(* Logix 5000 Rung export; software revision 16.05 *)

MODULES
   PBM : vendor None type None code None
   Local : vendor None type None code None
END_MODULES

TYPE ILX69PBM_STATUS_BACKPLANE :   // Backplane Block Status
STRUCT
   Input : ILX69PBM_STATUS_BACKPLANE_INPUT;
   Output : ILX69PBM_STATUS_BACKPLANE_OUTPUT;
END_STRUCT
END_TYPE

TYPE ILX69PBM_CONTROL_DPV1_WRITE_REQUEST :   // DPV1 Write Request
STRUCT
   Status : DINT;   // Status
   Command : DINT;   // Message Command. Set to 0x2212
   SlaveAddress : SINT;   // Slave Address
   SlotNumber : SINT;   // Slot Number
   Index : SINT;   // Index
   Length : SINT;   // Length
   Data : SINT[100];   // Write Data
END_STRUCT
END_TYPE

TYPE ILX69PBM_CONTROL_BACKPLANE :   // Backplane Block Control
STRUCT
   DisableAutoTransfer : BOOL;   // Disable Automatic Block Transfer
   Input : ILX69PBM_CONTROL_BACKPLANE_INPUT;
   Output : ILX69PBM_CONTROL_BACKPLANE_OUTPUT;
END_STRUCT
END_TYPE

TYPE ILX69PBM_UTIL_SLAVE_DIAG_COMMAND :   // Requested address for SlaveDiagnostic
STRUCT
   SlaveAddress : SINT;   // Slave Address
   DiagnosticMode : SINT;   // Diagnostic Mode
   Reserved1 : SINT;   // Reserved
   Reserved2 : SINT;   // Reserved
END_STRUCT
END_TYPE

TYPE ILX69PBM_CONTROL_BACKPLANE_OUTPUT :
STRUCT
   BlockID : SINT;   // Command Output Block Number. Use when DisableAutoTransfer is set.
   WriteBlock : BOOL;   // Send current commanded output block to module. Use when DisableAutoTransfer is set.
   CommitToProfibus : BOOL;   // Commit output block data to Profibus. Use when DisableAutoTransfer is set.
END_STRUCT
END_TYPE

TYPE ILX69PBM_UTIL_OUTPUT_ARRAY :
STRUCT
   DeviceCommandRegister : ILX69PBM_UTIL_DEV_COMMAND_REGISTER;   // Command Register
   DiagnosticSlaveAddress : ILX69PBM_UTIL_SLAVE_DIAG_COMMAND;   // Slave Address
   GlobalControlCommand : ILX69PBM_UTIL_GLOBAL_CONTROL_COMMAND;   // Global Control Command
   Reserved : SINT[4];   // Reserved
   OutputData : INT[240];   // PROFIBUS Output data.
END_STRUCT
END_TYPE

TYPE ILX69PBM_UTIL_GLOBAL_STATE_FIELD :   // PROFIBUS Master Global State Field
STRUCT
   ControlError : BOOL;   // Control error
   AutoClearError : BOOL;   // Auto clear error
   NonExchangeError : BOOL;   // Non exchange error
   FatalError : BOOL;   // Fatal error
   EventError : BOOL;   // Event error
   HostNotReady : BOOL;   // Host not ready notification
   Timeout : BOOL;   // Timeout
   Reserved1 : BOOL;   // Reserved
   MasterMainState : SINT;   // Master main state
   FaultySlaveAddress : SINT;   // Faulty remote address
   ErrorNumber : SINT;   // Error Number
   BusErrorCount : INT;   // Heavy bus error counter
   TimeoutCount : INT;   // Number of rejected PROFIBUS Telegr.
   Reserved : SINT[8];   // Reserved
   SlaveConfiguration : ILX69PBM_SLAVE128;   // Slave Config
   SlaveState : ILX69PBM_SLAVE128;   // Slave State
   SlaveDiagnostic : ILX69PBM_SLAVE128;   // Slave Diag
END_STRUCT
END_TYPE

TYPE ILX69PBM_UTIL_GLOBAL_CONTROL_COMMAND :   // Global Control Command
STRUCT
   SlaveAddress : SINT;   // Slave Address
   ControlCommand : SINT;   // Control Command to be sent
   GroupSelect : SINT;   // Group Select
   Reserved1 : SINT;   // Reserved
END_STRUCT
END_TYPE

TYPE ILX69PBM_CONTROL_DPV1_READ :   // DPV1 Read
STRUCT
   Initiate : BOOL;   // Initiate DPV1 Slave Read
   MSGStatus : ILX69PBM_MESSAGE_STATUS;   // Message Status
   Request : ILX69PBM_CONTROL_DPV1_READ_REQUEST;   // Request
   Response : ILX69PBM_CONTROL_DPV1_READ_RESPONSE;   // Response
END_STRUCT
END_TYPE

TYPE ILX69PBM_CONTROL_DPV1_WRITE :   // DPV1 Write
STRUCT
   Initiate : BOOL;   // Initiate DPV1 Slave Write
   MSGStatus : ILX69PBM_MESSAGE_STATUS;   // Message Status
   Request : ILX69PBM_CONTROL_DPV1_WRITE_REQUEST;   // Request
   Response : ILX69PBM_CONTROL_DPV1_WRITE_RESPONSE;   // Response
END_STRUCT
END_TYPE

TYPE ILX69PBM_CONTROL_SLAVECONTROLMSG :   // DPV0 Global Control
STRUCT
   Initiate : BOOL;   // Initiate Global Control
   MSGStatus : ILX69PBM_MESSAGE_STATUS;   // Message Status
   Request : ILX69PBM_CONTROL_SLAVECONTROLMSG_REQUEST;   // Request
   Response : ILX69PBM_CONTROL_SLAVECONTROLMSG_RESPONS;   // Response
END_STRUCT
END_TYPE

TYPE ILX69PBM_CONTROL_SLAVEDIAG_BLOCKRESPONSE :   // Slave Diagnostic Reponse
STRUCT
   SlaveAddress : SINT;   // Slave address
   SlaveDiagnosticFailure : SINT;   // Slave Diag Failure
   StationNotExist : BOOL;   // No response
   StationNotReady : BOOL;   // Station not ready
   ConfigurationFault : BOOL;   // Configuration faulty
   ExtendedDiagnostic : BOOL;   // Extended diagnostic
   SyncFreezeNoSupport : BOOL;   // Sync,Freeze not supported
   InvalidResponse : BOOL;   // Response faulty
   ParamterFault : BOOL;   // Parameters faulty
   MasterLock : BOOL;   // Locked by a master
   ParameterRequest : BOOL;   // Request new parameter
   StaticDiagnostic : BOOL;   // Static diagnostic
   Slave : BOOL;   // Set to 1 by a slave
   Watchdog : BOOL;   // Watchdog ON/OFF
   FreezeMode : BOOL;   // Freeze mode active
   SyncMode : BOOL;   // Sync mode active
   Reserved : BOOL;   // Reserved
   SlaveDeactivated : BOOL;   // Slave deactivated
   Reserved0 : BOOL;   // Reserved
   Reserved1 : BOOL;   // Reserved
   Reserved2 : BOOL;   // Reserved
   Reserved3 : BOOL;   // Reserved
   Reserved4 : BOOL;   // Reserved
   Reserved5 : BOOL;   // Reserved
   Reserved6 : BOOL;   // Reserved
   ExtendedDiagnosticOverflow : BOOL;   // Extended diagnostic overflow
   MasterAddress : SINT;   // Corresponding master address
   IdentNumber : INT;   // PROFIBUS Ident number
END_STRUCT
END_TYPE

TYPE ILX69PBM_CONTROL_DPV1_ALARM_RESPONSE :   // DPV1 Alarm Response Confirm
STRUCT
   Status : DINT;   // Status 0=OK
   Command : DINT;   // Should be 0x221D
   SlaveAddress : SINT;   // Slave Address
   AlarmType : SINT;   // Type of alarm received
   SlotNumber : SINT;   // Slot Number of module causing the alarm
   Specifier : SINT;   // Alarm specifier
   Function : SINT;   // Reserved
   ErrorDecode : SINT;   // 128 indicates DPV1 error
   ErrorCode1 : SINT;   // Error Code 1
   ErrorCode2 : SINT;   // Error Code 2
END_STRUCT
END_TYPE

TYPE ILX69PBM_STATUS_DPV1_ALARM_INDICATION :   // DPV1 Alarm Indication
STRUCT
   AlarmIndication : BOOL;   // Indicates an alarm
   AlarmOverrun : BOOL;   // Overflow of the modules internal alarm buffer
   AlarmIndicationCounter : SINT;   // Alarm indication counter
   SlaveAddress : SINT;   // Address of Slave with Alarm
   SlotNumber : SINT;   // Slot Number
   SequenceNumber : SINT;   // Sequence Number
   AlarmType : SINT;   // Alarm Type
   AlarmSpecification : SINT;   // Alarm Specification
END_STRUCT
END_TYPE

TYPE EDIT_ILX69PBM_DATA :   // Array size should be the same as the address table size in fdt Configuration Manager.
STRUCT
   INPUT : SINT[5712];   // Input Data
   OUTPUT : SINT[5760];   // Output Data
END_STRUCT
END_TYPE

TYPE ILX69PBM_STATUS_GLOBAL_STATE :   // Global State
STRUCT
   ControlError : BOOL;   // Control error. Parameterization error
   AutoClearError : BOOL;   // Auto clear error. Module stopped communication with all slaves and reached the auto-clear-end state.
   NonExchangeError : BOOL;   // Non exchange error. At least one slave has not reached the data exchange state and no process data will be exchanged.
   FatalError : BOOL;   // Fatal error. Because of major bus error, no further bus communication is possible.
   EventError : BOOL;   // Event error. Bus short circuits detected
   HostNotReady : BOOL;   // Host not ready notification. The Application program is not ready to communicate
   Timeout : BOOL;   // Timeout.Overstepped timeout supervision value because of rejected PROFIBUS telegrams.
   Reserved1 : BOOL;   // Reserved
   MasterMainState : SINT;   // Master main state. 00hex: OFFLINE 40hex: STOP 80hex: CLEAR C0hex: OPERATE
   FaultySlaveAddress : SINT;   // Faulty remote address. 0 ... 125 Error detected with a Slave device 255 Error with Master.
   ErrorNumber : SINT;   // Error Number. See Manual for details.
   BusErrorCount : INT;   // Heavy bus error counter
   TimeoutCount : INT;   // Number of rejected PROFIBUS Telegr.
   SlaveConfiguration : ILX69PBM_SLAVE128;   // Slave Config
   SlaveState : ILX69PBM_SLAVE128;   // Slave State
   SlaveDiagnostic : ILX69PBM_SLAVE128;   // Slave Diagnostic
END_STRUCT
END_TYPE

TYPE ILX69PBM_UTIL_INPUT_ARRAY :   // Input Array
STRUCT
   DeviceStatusRegister : ILX69PBM_UTIL_DEV_STATUS_REGISTER;   // Device Status
   FirmwareRevBPSize : ILX69PBM_UTIL_FW_REVISION_BPSIZE;   // Firmware Revision and Block Size
   GlobalStateField : ILX69PBM_UTIL_GLOBAL_STATE_FIELD;   // Global State Field
   SlaveDiagnostic : ILX69PBM_UTIL_SLAVE_DIAG_DATA;   // Slave Diagnostic
   DPV1AlarmIndication : ILX69PBM_UTIL_DPV1_ALARM_INDICATION;   // DPV1 Alarm Indication
   InputData : INT[204];   // PROFIBUS Input data.
END_STRUCT
END_TYPE

TYPE ILX69PBM_UTIL_CONFIG :   // Control
STRUCT
   MaxBlockTransferOut : SINT;   // Maximum Block Number Out. Calculated by total output bytes divided by 480.
   MaxBlockTransferIn : SINT;   // Maximum Block Number In. Calculated by total input bytes divided by 408.
   MaxBlockDataOut : SINT;
END_STRUCT
END_TYPE

TYPE ILX69PBM_CONTROL_DPV1_READ_RESPONSE :   // DPV1 Read Response
STRUCT
   Status : DINT;   // Status
   Command : DINT;   // Should be 0x2211
   SlaveAddress : SINT;   // Slave Address
   SlotNumber : SINT;   // Slot Number
   Index : SINT;   // Index
   Length : SINT;   // Length
   Data : SINT[100];   // Data or Error Codes (first 2 bytes)
END_STRUCT
END_TYPE

TYPE ILX69PBM_CONTROL_DPV1_ALARM :   // Alarm Response
STRUCT
   Initiate : BOOL;   // Initiate DPV1 Alarm Response
   MSGStatus : ILX69PBM_MESSAGE_STATUS;   // Message Status
   Request : ILX69PBM_CONTROL_DPV1_ALARM_REQUEST;   // Request
   Response : ILX69PBM_CONTROL_DPV1_ALARM_RESPONSE;   // Response
END_STRUCT
END_TYPE

TYPE ILX69PBM_CONTROL_SLAVECONTROLBLOCK :
STRUCT
   Initiate : BOOL;   // Initiate Slave Control
   Address : SINT;   // Slave Address
   MSGStatus : ILX69PBM_MESSAGE_STATUS;   // Message Status
   SlaveCommand : ILX69PBM_CONTROL_SLAVECONTROLBLOCK_CMD;   // Slave Control Command
END_STRUCT
END_TYPE

TYPE ILX69PBM_MODULEDEF :   // ILX69-PBM PROFIBUS Master Module Definition
STRUCT
   DATA : EDIT_ILX69PBM_DATA;   // Data
   STATUS : ILX69PBM_STATUS;   // Module Status
   CONTROL : ILX69PBM_CONTROL;   // Module Control
END_STRUCT
END_TYPE

TYPE ILX69PBM_UTIL_SLAVE_DIAG_DATA :   // Slave standard diagnostic data according to PROFIBUS norm.
STRUCT
   SlaveAddress : SINT;   // Slave address
   SlaveDiagnosticFailure : SINT;   // Slave Diag Failure
   Sta1_StationNotExist : BOOL;   // No response
   Sta1_StationNotReady : BOOL;   // Station not ready
   Sta1_ConfigurationFault : BOOL;   // Configuration faulty
   Sta1_ExtendedDiagnostic : BOOL;   // Extended diagnostic
   Sta1_SyncFreezeNoSupport : BOOL;   // Sync,Freeze not supported
   Sta1_InvalidResponse : BOOL;   // Response faulty
   Sta1_ParamterFault : BOOL;   // Parameters faulty
   Sta1_MasterLock : BOOL;   // Locked by a master
   Sta2_ParameterRequest : BOOL;   // Request new parameter
   Sta2_StaticDiagnostic : BOOL;   // Static diagnostic
   Sta2_Slave : BOOL;   // Set to 1 by a slave
   Sta2_Watchdog : BOOL;   // Watchdog ON/OFF
   Sta2_FreezeMode : BOOL;   // Freeze mode active
   Sta2_SyncMode : BOOL;   // Sync mode active
   Sta2_Reserved : BOOL;   // Reserved
   Sta2_SlaveDeactivated : BOOL;   // Slave deactivated
   Sta3_Reserved0 : BOOL;   // Reserved
   Sta3_Reserved1 : BOOL;   // Reserved
   Sta3_Reserved2 : BOOL;   // Reserved
   Sta3_Reserved3 : BOOL;   // Reserved
   Sta3_Reserved4 : BOOL;   // Reserved
   Sta3_Reserved5 : BOOL;   // Reserved
   Sta3_Reserved6 : BOOL;   // Reserved
   Sta3_ExtendedDiagnosticOverflow : BOOL;   // Extended diagnostic overflow
   MasterAddress : SINT;   // Corresponding master address
   IdentNumber : INT;   // PROFIBUS Ident number
END_STRUCT
END_TYPE

TYPE ILX69PBM_STATUS :   // Status
STRUCT
   Communication : BOOL;   // Profibus communication is started and the module is engaged in cyclic data exchange with at least one Slave
   Running : BOOL;   // Running. Module is ready for communication.
   Ready : BOOL;   // Ready. Module is operational.
   FirmwareRevision : ILX69PBM_STATUS_FW_REVISION;   // Firmware Revision
   GlobalState : ILX69PBM_STATUS_GLOBAL_STATE;   // Global State
   DPV1AlarmIndication : ILX69PBM_STATUS_DPV1_ALARM_INDICATION;   // DPV1 Alarm Indication
   BackplaneBlock : ILX69PBM_STATUS_BACKPLANE;   // Backplane Block Status
END_STRUCT
END_TYPE

TYPE ILX69PBM_CONTROL_SLAVECONTROLMSG_CMD :   // Slave Control Message Command
STRUCT
   UnFreeze : BOOL;   // Unfreeze Input Data
   Freeze : BOOL;   // Freeze Input Data
   UnSync : BOOL;   // Neutralize the sync command or Unsync
   Sync : BOOL;   // Freeze Output Data until sync command is neutralized
   GroupSelect : SINT;   // Group Select
END_STRUCT
END_TYPE

TYPE ILX69PBM_CONTROL_SLAVECONTROLBLOCK_CMD :   // Slave Control Block Command
STRUCT
   ClearData : BOOL;   // Clear Output Data
   UnFreeze : BOOL;   // Unfreeze Input Data
   Freeze : BOOL;   // Freeze Input Data
   UnSync : BOOL;   // Neutralize the sync command or Unsync
   Sync : BOOL;   // Freeze Output Data until sync command is neutralized
   GroupSelect : SINT;   // Group Select
END_STRUCT
END_TYPE

TYPE ILX69PBM_UTIL_DPV1_ALARM_INDICATION :   // DPV1 Alarm Indication
STRUCT
   AlarmIndication : BOOL;   // Indicates an alarm
   Reserved1 : BOOL;   // Reserved
   Reserved2 : BOOL;   // Reserved
   Reserved3 : BOOL;   // Reserved
   Reserved4 : BOOL;   // Reserved
   Reserved5 : BOOL;   // Reserved
   Reserved6 : BOOL;   // Reserved
   AlarmOverrun : BOOL;   // Overflow of the modules internal alarm buffer
   AlarmIndicationCounter : SINT;   // Alarm indication counter
   SlaveAddress : SINT;   // Address of Slave with Alarm
   SlotNumber : SINT;   // Slot Number
   SequenceNumber : SINT;   // Sequence Number
   AlarmType : SINT;   // Alarm Type
   AlarmSpecification : SINT;   // Alarm Specification
   Reserved7 : SINT;   // Reserved
END_STRUCT
END_TYPE

TYPE ILX69PBM_CONTROL_SLAVEDIAG_EXT :   // Slave Extended Diagnostic Data
STRUCT
   Initiate : BOOL;   // Initiate Slave Extended Diagnostic
   MSGStatus : ILX69PBM_MESSAGE_STATUS;   // Message Status
   Request : ILX69PBM_CONTROL_SLAVEDIAG_EXT_REQUEST;   // Request
   Response : ILX69PBM_CONTROL_SLAVEDIAG_EXT_RESPONSE;   // Reponse
END_STRUCT
END_TYPE

TYPE ILX69PBM_CONTROL_SLAVEDIAG_EXT_REQUEST :   // Slave Extended Diagnostic Request
STRUCT
   Status : DINT;   // Slave Status
   Command : DINT;   // Message Command. Set to 0x220a
   Address : DINT;   // Slave Address
   Flag : DINT;   // Flag
END_STRUCT
END_TYPE

TYPE ILX69PBM_UTIL_DEV_COMMAND_REGISTER :   // Device Command Register
STRUCT
   Reserved0 : BOOL;   // Reserved
   Reserved1 : BOOL;   // Reserved
   Reserved2 : BOOL;   // Reserved
   Reserved3 : BOOL;   // Reserved
   Reserved4 : BOOL;   // Reserved
   NotReady : BOOL;   // Application Not Ready
   Reserved5 : BOOL;   // Init ( Warm boot )
   Reset : BOOL;   // Reset ( Cold boot )
   HsReq0 : BOOL;   // Slave Diag Request
   HsReq1 : BOOL;   // Global Control Request
   HsReq2 : BOOL;   // Reserved
   HsReq3 : BOOL;   // Reserved
   HsReq4 : BOOL;   // Reserved
   HsReq5 : BOOL;   // Reserved
   HsReq6 : BOOL;   // Reserved
   HsReq7 : BOOL;   // Reserved
   BlockTransferOut : SINT;   // Reserved
   BlockTransferIn : SINT;   // Reserved
END_STRUCT
END_TYPE

TYPE ILX69PBM_STATUS_BACKPLANE_INPUT :   // Input Block Status
STRUCT
   ReturnedBlockID : SINT;   // Current Input block of module.
   BlockRead : BOOL;   // The requested block has been transferred to Data.Input Array with appropriate offset.
END_STRUCT
END_TYPE

TYPE ILX69PBM_STATUS_BACKPLANE_OUTPUT :   // Output Block Status
STRUCT
   CommittedToProfibus : BOOL;   // Output Data is committed to Profibus
   CurrentBlockToModule : BOOL;   // The current output block data is sent to the module but not committed to Profibus (if not block 0).
   BlockID : SINT;   // Current Output block of module.
END_STRUCT
END_TYPE

TYPE ILX69PBM_CONTROL_SLAVEDIAG_EXT_RESPONSE :   // Slave Extented Diagnostic Response
STRUCT
   Status : DINT;   // Status 0=OK
   Command : DINT;   // Should return 0x220A
   SlaveAddress : DINT;   // Slave Address
   Diagnostic : SINT[256];   // Slave Diagnostic
END_STRUCT
END_TYPE

TYPE ILX69PBM_UTIL_FW_REVISION_BPSIZE :   // Firmware Major/Minor Revision and Block Plane Size
STRUCT
   FwMinor : SINT;   // Firmware Minor Revison
   FwMajor : SINT;   // Firmware Major Revison
   Input : SINT;   // Number of Blocks required to transfer all Profibus cyclic Input data.
   Output : SINT;   // Number of Blocks required to transfer all Profibus cyclic Output data.
END_STRUCT
END_TYPE

TYPE ILX69PBM_CONTROL_DPV1 :   // DPV1
STRUCT
   Read : ILX69PBM_CONTROL_DPV1_READ;   // DPV1 Read Request
   Write : ILX69PBM_CONTROL_DPV1_WRITE;   // DPV1 Write Request
   Alarm : ILX69PBM_CONTROL_DPV1_ALARM;   // DPV1 Alarm Response Request
END_STRUCT
END_TYPE

TYPE ILX69PBM_UTIL_DEV_STATUS_REGISTER :   // Device Status Register
STRUCT
   Reserved0 : BOOL;   // Reserved
   Reserved1 : BOOL;   // Reserved
   Reserved2 : BOOL;   // Reserved
   Reserved3 : BOOL;   // Reserved
   Reserved4 : BOOL;   // Reserved
   Communication : BOOL;   // Communication
   Running : BOOL;   // Running
   Ready : BOOL;   // Ready
   HsAck0 : BOOL;   // Slave Diag Acknowledge
   HsAck1 : BOOL;   // Global Control Acknowledge
   HsAck2 : BOOL;
   HsAck3 : BOOL;
   HsAck4 : BOOL;
   HsAck5 : BOOL;
   HsAck6 : BOOL;
   HsAck7 : BOOL;
   BlockTransferOut : SINT;
   BlockTransferIn : SINT;
END_STRUCT
END_TYPE

TYPE ILX69PBM_CONTROL_DPV1_READ_REQUEST :   // DPV1 Read Request
STRUCT
   Status : DINT;   // Status
   Command : DINT;   // Message Command. Set to 0x2210
   SlaveAddress : SINT;   // Slave Address
   SlotNumber : SINT;   // Slot Number
   Index : SINT;   // Index
   Length : SINT;   // Length
END_STRUCT
END_TYPE

TYPE ILX69PBM_CONTROL_BACKPLANE_INPUT :
STRUCT
   BlockID : SINT;   // Requested Input Block Number. Use when DisableAutoTransfer is set.
   ReadBlock : BOOL;   // Initiate to receive the data from the requested Input Block Number. Use when DisableAutoTransfer is set.
END_STRUCT
END_TYPE

TYPE ILX69PBM_CONTROL_SLAVECONTROL :   // Cyclic Slave Control
STRUCT
   SetSlaveControl : ILX69PBM_CONTROL_SLAVECONTROLBLOCK;   // Slave Control via Block Transfer
   SetSlaveControl_MSG : ILX69PBM_CONTROL_SLAVECONTROLMSG;   // Slave Global Control via MSG
END_STRUCT
END_TYPE

TYPE ILX69PBM_CONTROL_SLAVECONTROLMSG_REQUEST :   // Global Control Request
STRUCT
   Status : DINT;   // Status
   Command : DINT;   // Message Command. Set to 0x2220
   Address : DINT;   // Slave Address
   Reserved : ILX69PBM_CONTROL_SLAVECONTROLMSG_RSVD;   // Reserved
   SlaveCommand : ILX69PBM_CONTROL_SLAVECONTROLMSG_CMD;   // Slave Command
END_STRUCT
END_TYPE

TYPE ILX69PBM_CONTROL_DPV1_ALARM_REQUEST :   // DPV1 Alarm Response Request
STRUCT
   Status : DINT;   // Status
   Command : DINT;   // Message Command. Set to 0x221C
   SlaveAddress : SINT;   // Slave Address
   AlarmType : SINT;   // Type of the received alarm
   SlotNumber : SINT;   // Slot number of module causing the alarm
   Specifier : SINT;   // Alarm specifier
   Function : SINT;   // Reserved
   Reserved : SINT[3];   // Reserved
END_STRUCT
END_TYPE

TYPE ILX69PBM_CONTROL_SLAVECONTROLMSG_RESPONS :   // DPV0 Slave Global Control Confirm
STRUCT
   Status : DINT;   // Status 0=OK
   Command : DINT;   // Should return 0x2221
END_STRUCT
END_TYPE

TYPE ILX69PBM_CONTROL_SLAVECONTROLMSG_RSVD :
STRUCT
   SyncCommand : DINT;   // Sync Command
   FreezeCommand : DINT;   // Freeze Command
   GroupSelect : DINT;   // Group selection
END_STRUCT
END_TYPE

TYPE ILX69PBM_CONTROL_SLAVEDIAG :   // Diagnostic Data
STRUCT
   GetSlaveDiag : ILX69PBM_CONTROL_SLAVEDIAG_BLOCK;   // Slave Diagnostic Data via Block Transfer
   GetSlaveDiagExtended_MSG : ILX69PBM_CONTROL_SLAVEDIAG_EXT;   // Slave Extended Diagnostic via MSG
END_STRUCT
END_TYPE

TYPE ILX69PBM_STATUS_FW_REVISION :   // Firmware Major/Minor Revision
STRUCT
   FwMinor : SINT;   // Firmware Minor Revison
   FwMajor : SINT;   // Firmware Major Revison
END_STRUCT
END_TYPE

TYPE ILX69PBM_CONTROL_DPV1_WRITE_RESPONSE :   // DPV1 Write Response
STRUCT
   Status : DINT;   // Status 0=OK
   Command : DINT;   // Should return 0x2213
   SlaveAddress : SINT;   // Slave Address
   SlotNumber : SINT;   // Slot Number
   Index : SINT;   // Index
   Length : SINT;   // Length
   ErrorDecode : SINT;   // Error 128=DPV1 error
   ErrorCode1 : SINT;   // Error Code 1
   ErrorCode2 : SINT;   // Error Code 2
   Reserved : SINT;   // Reserved
END_STRUCT
END_TYPE

TYPE ILX69PBM_SLAVE128 :
STRUCT
   Slave : BOOL[128];   // Slave
END_STRUCT
END_TYPE

TYPE ILX69PBM_CONTROL_SLAVEDIAG_BLOCK :   // Slave Diagnostic Data
STRUCT
   Initiate : BOOL;   // Initiate Slave Diagnostic
   Address : SINT;   // Slave Address
   Function : SINT;   // Function: 0-Requested from Master 1-Requested from Slave
   MSGStatus : ILX69PBM_MESSAGE_STATUS;   // Message Status
   Response : ILX69PBM_CONTROL_SLAVEDIAG_BLOCKRESPONSE;   // Diagnostic Response
END_STRUCT
END_TYPE

TYPE ILX69PBM_CONTROL :
STRUCT
   DisableProfibus : BOOL;   // Halt Profibus Communication
   ColdBoot : BOOL;   // Cold Boot Reset
   BackplaneBlock : ILX69PBM_CONTROL_BACKPLANE;   // Block Control
   DPV1 : ILX69PBM_CONTROL_DPV1;   // DPV1 Data
   SlaveDiagnostic : ILX69PBM_CONTROL_SLAVEDIAG;   // Slave Diagnostic Data
   SlaveControl : ILX69PBM_CONTROL_SLAVECONTROL;   // Slave Control
END_STRUCT
END_TYPE

TYPE ILX69PBM_MESSAGE_STATUS :   // Message Status
STRUCT
   Done : BOOL;   // Message transmitted. Response is available
   Error : BOOL;   // Last message transmitted with an error
   DoneCount : DINT;   // Response OK Count
   ErrorCount : DINT;   // Error Count
END_STRUCT
END_TYPE

TYPE ILX69PBM_UTIL :
STRUCT
   InputArray : ILX69PBM_UTIL_INPUT_ARRAY;   // Input from Module
   OutputArray : ILX69PBM_UTIL_OUTPUT_ARRAY;   // Output to Module
   InputOffset : INT;
   OutputOffset : INT;
   InputSize : INT;
   OutputSize : INT;
   InputDataSize : INT;
   InputCopyLength : INT;
   OutputDataSize : INT;
   OutputCopyLength : INT;
   OutputCopyLastLength : INT;
   OutputConnectionSize : INT;
   UTILOutputCopyLength : INT;
   SlaveDiagErrorTimer : TIMER;
   SlaveControlErrorTimer : TIMER;
   Config : ILX69PBM_UTIL_CONFIG;
END_STRUCT
END_TYPE

ADD_ON_INSTRUCTION AOIILX69PBM   (* revision 1.9, vendor ProSoft Technology Inc., ExecutePrescan *)
// Add-On instruction for ILX69-PBM ProSoft module
// Revision note:
// V1.9 Unlocked AOI
// V1.8 Moved FLL UTIL.Output Array
// V1.7 Use local BlockID increment latch
// V1.6 Clear AOI UTIL local tag
VAR_IN_OUT
   ILX69PBM : ILX69PBM_MODULEDEF; {required}
   Connection_Input : INT[248]; {required}
        [0].5   // Communication
        [0].6   // Running
        [0].7   // Ready
   Connection_Output : INT[248]; {required}
   MSGSlaveDiagRequest : MESSAGE; {required}   // Slave Diagnostic Request Message
   MSGGlobalControl : MESSAGE; {required}   // Slave Global Control Message
   MSGDPV1Read : MESSAGE; {required}   // DPV1 Read Message
   MSGDPV1Write : MESSAGE; {required}   // DPV1 Write Message
   MSGDPV1Alarm : MESSAGE; {required}   // DPV1 Alarm Response Message
END_VAR
VAR
   UTIL : ILX69PBM_UTIL;
   InputBlockIDIncrementComplete : BOOL;
END_VAR

ROUTINE Logic   (* ladder *)
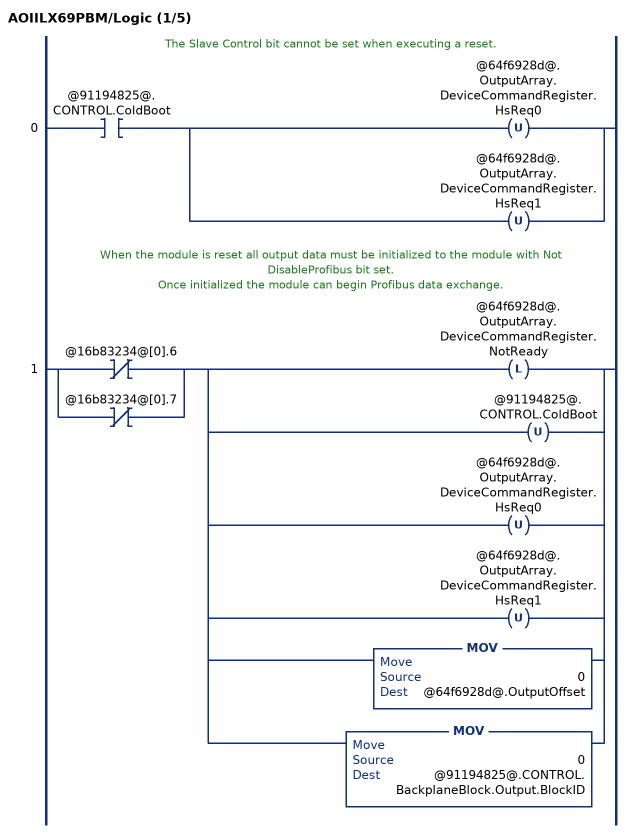
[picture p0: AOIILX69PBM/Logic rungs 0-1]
   // The Slave Control bit cannot be set when executing a reset.
   0: XIC(@91194825@.CONTROL.ColdBoot)[OTU(@64f6928d@.OutputArray.DeviceCommandRegister.HsReq0) ,OTU(@64f6928d@.OutputArray.DeviceCommandRegister.HsReq1) ];
   // When the module is reset all output data must be initialized to the module with Not DisableProfibus bit set.
   // Once initialized the module can begin Profibus data exchange.
   1: [XIO(@16b83234@[0].6) ,XIO(@16b83234@[0].7) ][OTL(@64f6928d@.OutputArray.DeviceCommandRegister.NotReady) ,OTU(@91194825@.CONTROL.ColdBoot) ,OTU(@64f6928d@.OutputArray.DeviceCommandRegister.HsReq0) ,OTU(@64f6928d@.OutputArray.DeviceCommandRegister.HsReq1) ,MOV(0,@64f6928d@.OutputOffset) ,MOV(0,@91194825@.CONTROL.BackplaneBlock.Output.BlockID) ];
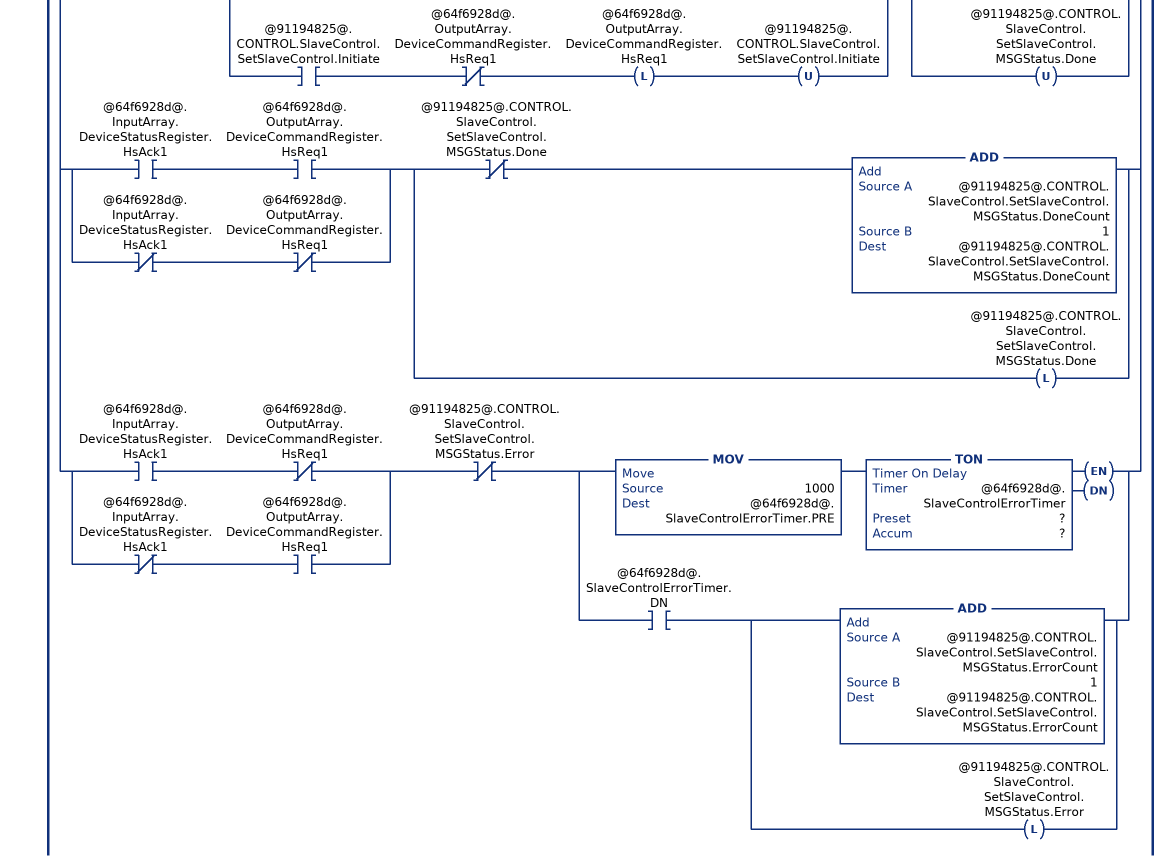
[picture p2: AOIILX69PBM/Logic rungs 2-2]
   // Handle Block Slave Diagnostic and Control
   2: [[XIC(@91194825@.CONTROL.SlaveDiagnostic.GetSlaveDiag.Initiate) [XIC(@64f6928d@.OutputArray.DeviceCommandRegister.HsReq0) OTU(@64f6928d@.OutputArray.DeviceCommandRegister.HsReq0) OTU(@91194825@.CONTROL.SlaveDiagnostic.GetSlaveDiag.Initiate) ,XIC(@91194825@.CONTROL.SlaveDiagnostic.GetSlaveDiag.Initiate) XIO(@64f6928d@.OutputArray.DeviceCommandRegister.HsReq0) OTL(@64f6928d@.OutputArray.DeviceCommandRegister.HsReq0) OTU(@91194825@.CONTROL.SlaveDiagnostic.GetSlaveDiag.Initiate) ] [OTU(@91194825@.CONTROL.SlaveDiagnostic.GetSlaveDiag.MSGStatus.Error) ,OTU(@91194825@.CONTROL.SlaveDiagnostic.GetSlaveDiag.MSGStatus.Done) ] ,[[XIC(@64f6928d@.InputArray.DeviceStatusRegister.HsAck0) XIC(@64f6928d@.OutputArray.DeviceCommandRegister.HsReq0) ,XIO(@64f6928d@.InputArray.DeviceStatusRegister.HsAck0) XIO(@64f6928d@.OutputArray.DeviceCommandRegister.HsReq0) ] [XIO(@91194825@.CONTROL.SlaveDiagnostic.GetSlaveDiag.MSGStatus.Done) ADD(@91194825@.CONTROL.SlaveDiagnostic.GetSlaveDiag.MSGStatus.DoneCount,1,@91194825@.CONTROL.SlaveDiagnostic.GetSlaveDiag.MSGStatus.DoneCount) ,OTL(@91194825@.CONTROL.SlaveDiagnostic.GetSlaveDiag.MSGStatus.Done) ] ,[XIC(@64f6928d@.InputArray.DeviceStatusRegister.HsAck0) XIO(@64f6928d@.OutputArray.DeviceCommandRegister.HsReq0) ,XIO(@64f6928d@.InputArray.DeviceStatusRegister.HsAck0) XIC(@64f6928d@.OutputArray.DeviceCommandRegister.HsReq0) ] XIO(@91194825@.CONTROL.SlaveDiagnostic.GetSlaveDiag.MSGStatus.Error) [MOV(1000,@64f6928d@.SlaveDiagErrorTimer.PRE) TON(@64f6928d@.SlaveDiagErrorTimer,?,?) ,XIC(@64f6928d@.SlaveDiagErrorTimer.DN) [ADD(@91194825@.CONTROL.SlaveDiagnostic.GetSlaveDiag.MSGStatus.ErrorCount,1,@91194825@.CONTROL.SlaveDiagnostic.GetSlaveDiag.MSGStatus.ErrorCount) ,OTL(@91194825@.CONTROL.SlaveDiagnostic.GetSlaveDiag.MSGStatus.Error) ] ] ] ] ,[XIC(@91194825@.CONTROL.SlaveControl.SetSlaveControl.Initiate) [XIC(@64f6928d@.OutputArray.DeviceCommandRegister.HsReq1) OTU(@64f6928d@.OutputArray.DeviceCommandRegister.HsReq1) OTU(@91194825@.CONTROL.SlaveControl.SetSlaveControl.Initiate) ,XIC(@91194825@.CONTROL.SlaveControl.SetSlaveControl.Initiate) XIO(@64f6928d@.OutputArray.DeviceCommandRegister.HsReq1) OTL(@64f6928d@.OutputArray.DeviceCommandRegister.HsReq1) OTU(@91194825@.CONTROL.SlaveControl.SetSlaveControl.Initiate) ] [OTU(@91194825@.CONTROL.SlaveControl.SetSlaveControl.MSGStatus.Error) ,OTU(@91194825@.CONTROL.SlaveControl.SetSlaveControl.MSGStatus.Done) ] ,[[XIC(@64f6928d@.InputArray.DeviceStatusRegister.HsAck1) XIC(@64f6928d@.OutputArray.DeviceCommandRegister.HsReq1) ,XIO(@64f6928d@.InputArray.DeviceStatusRegister.HsAck1) XIO(@64f6928d@.OutputArray.DeviceCommandRegister.HsReq1) ] [XIO(@91194825@.CONTROL.SlaveControl.SetSlaveControl.MSGStatus.Done) ADD(@91194825@.CONTROL.SlaveControl.SetSlaveControl.MSGStatus.DoneCount,1,@91194825@.CONTROL.SlaveControl.SetSlaveControl.MSGStatus.DoneCount) ,OTL(@91194825@.CONTROL.SlaveControl.SetSlaveControl.MSGStatus.Done) ] ,[XIC(@64f6928d@.InputArray.DeviceStatusRegister.HsAck1) XIO(@64f6928d@.OutputArray.DeviceCommandRegister.HsReq1) ,XIO(@64f6928d@.InputArray.DeviceStatusRegister.HsAck1) XIC(@64f6928d@.OutputArray.DeviceCommandRegister.HsReq1) ] XIO(@91194825@.CONTROL.SlaveControl.SetSlaveControl.MSGStatus.Error) [MOV(1000,@64f6928d@.SlaveControlErrorTimer.PRE) TON(@64f6928d@.SlaveControlErrorTimer,?,?) ,XIC(@64f6928d@.SlaveControlErrorTimer.DN) [ADD(@91194825@.CONTROL.SlaveControl.SetSlaveControl.MSGStatus.ErrorCount,1,@91194825@.CONTROL.SlaveControl.SetSlaveControl.MSGStatus.ErrorCount) ,OTL(@91194825@.CONTROL.SlaveControl.SetSlaveControl.MSGStatus.Error) ] ] ] ] ];
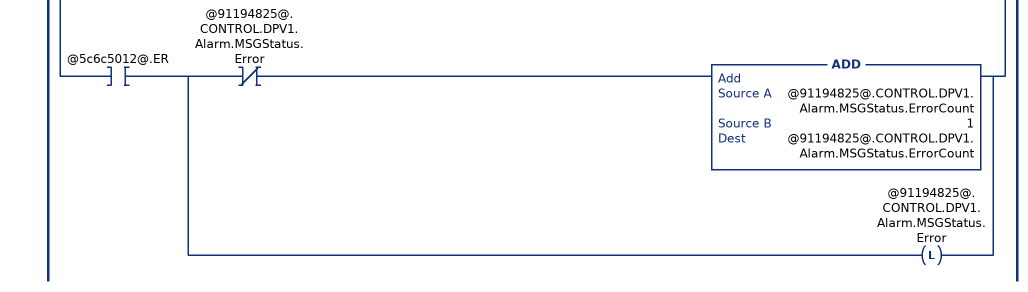
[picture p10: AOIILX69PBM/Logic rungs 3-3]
   // Message Handling
   3: [[XIC(@91194825@.CONTROL.SlaveDiagnostic.GetSlaveDiagExtended_MSG.Initiate) [MOV(8714,@91194825@.CONTROL.SlaveDiagnostic.GetSlaveDiagExtended_MSG.Request.Command) ,MSG(@9c913fae@) ,OTU(@91194825@.CONTROL.SlaveDiagnostic.GetSlaveDiagExtended_MSG.Initiate) ,OTU(@91194825@.CONTROL.SlaveDiagnostic.GetSlaveDiagExtended_MSG.MSGStatus.Error) ,OTU(@91194825@.CONTROL.SlaveDiagnostic.GetSlaveDiagExtended_MSG.MSGStatus.Done) ] ,XIC(@9c913fae@.DN) [XIO(@91194825@.CONTROL.SlaveDiagnostic.GetSlaveDiagExtended_MSG.MSGStatus.Done) ADD(@91194825@.CONTROL.SlaveDiagnostic.GetSlaveDiagExtended_MSG.MSGStatus.DoneCount,1,@91194825@.CONTROL.SlaveDiagnostic.GetSlaveDiagExtended_MSG.MSGStatus.DoneCount) ,OTL(@91194825@.CONTROL.SlaveDiagnostic.GetSlaveDiagExtended_MSG.MSGStatus.Done) ] ,XIC(@9c913fae@.ER) [XIO(@91194825@.CONTROL.SlaveDiagnostic.GetSlaveDiagExtended_MSG.MSGStatus.Error) ADD(@91194825@.CONTROL.SlaveDiagnostic.GetSlaveDiagExtended_MSG.MSGStatus.ErrorCount,1,@91194825@.CONTROL.SlaveDiagnostic.GetSlaveDiagExtended_MSG.MSGStatus.ErrorCount) ,OTL(@91194825@.CONTROL.SlaveDiagnostic.GetSlaveDiagExtended_MSG.MSGStatus.Error) ] ] ,[XIC(@91194825@.CONTROL.SlaveControl.SetSlaveControl_MSG.Initiate) [MOV(8736,@91194825@.CONTROL.SlaveControl.SetSlaveControl_MSG.Request.Command) ,[XIC(@91194825@.CONTROL.SlaveControl.SetSlaveControl_MSG.Request.SlaveCommand.UnFreeze) MVM(4,4,@91194825@.CONTROL.SlaveControl.SetSlaveControl_MSG.Request.Reserved.FreezeCommand) ,XIO(@91194825@.CONTROL.SlaveControl.SetSlaveControl_MSG.Request.SlaveCommand.UnFreeze) MVM(0,4,@91194825@.CONTROL.SlaveControl.SetSlaveControl_MSG.Request.Reserved.FreezeCommand) ] ,[XIC(@91194825@.CONTROL.SlaveControl.SetSlaveControl_MSG.Request.SlaveCommand.Freeze) MVM(8,8,@91194825@.CONTROL.SlaveControl.SetSlaveControl_MSG.Request.Reserved.FreezeCommand) ,XIO(@91194825@.CONTROL.SlaveControl.SetSlaveControl_MSG.Request.SlaveCommand.Freeze) MVM(0,8,@91194825@.CONTROL.SlaveControl.SetSlaveControl_MSG.Request.Reserved.FreezeCommand) ] ,[XIC(@91194825@.CONTROL.SlaveControl.SetSlaveControl_MSG.Request.SlaveCommand.UnSync) MVM(16#10,16#10,@91194825@.CONTROL.SlaveControl.SetSlaveControl_MSG.Request.Reserved.SyncCommand) ,XIO(@91194825@.CONTROL.SlaveControl.SetSlaveControl_MSG.Request.SlaveCommand.UnSync) MVM(0,16#10,@91194825@.CONTROL.SlaveControl.SetSlaveControl_MSG.Request.Reserved.SyncCommand) ] ,[XIC(@91194825@.CONTROL.SlaveControl.SetSlaveControl_MSG.Request.SlaveCommand.Sync) MVM(16#20,16#20,@91194825@.CONTROL.SlaveControl.SetSlaveControl_MSG.Request.Reserved.SyncCommand) ,XIO(@91194825@.CONTROL.SlaveControl.SetSlaveControl_MSG.Request.SlaveCommand.Sync) MVM(0,16#20,@91194825@.CONTROL.SlaveControl.SetSlaveControl_MSG.Request.Reserved.SyncCommand) ] ,MOV(@91194825@.CONTROL.SlaveControl.SetSlaveControl_MSG.Request.SlaveCommand.GroupSelect,@91194825@.CONTROL.SlaveControl.SetSlaveControl_MSG.Request.Reserved.GroupSelect) ,MSG(@5cc5b539@) ,OTU(@91194825@.CONTROL.SlaveControl.SetSlaveControl_MSG.Initiate) ,OTU(@91194825@.CONTROL.SlaveControl.SetSlaveControl_MSG.MSGStatus.Error) ,OTU(@91194825@.CONTROL.SlaveControl.SetSlaveControl_MSG.MSGStatus.Done) ] ,XIC(@5cc5b539@.DN) [XIO(@91194825@.CONTROL.SlaveControl.SetSlaveControl_MSG.MSGStatus.Done) ADD(@91194825@.CONTROL.SlaveControl.SetSlaveControl_MSG.MSGStatus.DoneCount,1,@91194825@.CONTROL.SlaveControl.SetSlaveControl_MSG.MSGStatus.DoneCount) ,OTL(@91194825@.CONTROL.SlaveControl.SetSlaveControl_MSG.MSGStatus.Done) ] ,XIC(@5cc5b539@.ER) [XIO(@91194825@.CONTROL.SlaveControl.SetSlaveControl_MSG.MSGStatus.Error) ADD(@91194825@.CONTROL.SlaveControl.SetSlaveControl_MSG.MSGStatus.ErrorCount,1,@91194825@.CONTROL.SlaveControl.SetSlaveControl_MSG.MSGStatus.ErrorCount) ,OTL(@91194825@.CONTROL.SlaveControl.SetSlaveControl_MSG.MSGStatus.Error) ] ] ,[XIC(@91194825@.CONTROL.DPV1.Read.Initiate) [MOV(8720,@91194825@.CONTROL.DPV1.Read.Request.Command) ,MSG(@2c4ca778@) ,OTU(@91194825@.CONTROL.DPV1.Read.Initiate) ,OTU(@91194825@.CONTROL.DPV1.Read.MSGStatus.Error) ,OTU(@91194825@.CONTROL.DPV1.Read.MSGStatus.Done) ] ,XIC(@2c4ca778@.DN) [XIO(@91194825@.CONTROL.DPV1.Read.MSGStatus.Done) ADD(@91194825@.CONTROL.DPV1.Read.MSGStatus.DoneCount,1,@91194825@.CONTROL.DPV1.Read.MSGStatus.DoneCount) ,OTL(@91194825@.CONTROL.DPV1.Read.MSGStatus.Done) ] ,XIC(@2c4ca778@.ER) [XIO(@91194825@.CONTROL.DPV1.Read.MSGStatus.Error) ADD(@91194825@.CONTROL.DPV1.Read.MSGStatus.ErrorCount,1,@91194825@.CONTROL.DPV1.Read.MSGStatus.ErrorCount) ,OTL(@91194825@.CONTROL.DPV1.Read.MSGStatus.Error) ] ] ,[XIC(@91194825@.CONTROL.DPV1.Write.Initiate) [CPT(@c5f8241b@.REQ_LEN,12+@91194825@.CONTROL.DPV1.Write.Request.Length) [LES(@c5f8241b@.REQ_LEN,12) MOV(12,@c5f8241b@.REQ_LEN) ,GRT(@c5f8241b@.REQ_LEN,112) MOV(112,@c5f8241b@.REQ_LEN) ] ,MOV(8722,@91194825@.CONTROL.DPV1.Write.Request.Command) ,MSG(@c5f8241b@) ,OTU(@91194825@.CONTROL.DPV1.Write.Initiate) ,OTU(@91194825@.CONTROL.DPV1.Write.MSGStatus.Error) ,OTU(@91194825@.CONTROL.DPV1.Write.MSGStatus.Done) ] ,XIC(@c5f8241b@.DN) [XIO(@91194825@.CONTROL.DPV1.Write.MSGStatus.Done) ADD(@91194825@.CONTROL.DPV1.Write.MSGStatus.DoneCount,1,@91194825@.CONTROL.DPV1.Write.MSGStatus.DoneCount) ,OTL(@91194825@.CONTROL.DPV1.Write.MSGStatus.Done) ] ,XIC(@c5f8241b@.ER) [XIO(@91194825@.CONTROL.DPV1.Write.MSGStatus.Error) ADD(@91194825@.CONTROL.DPV1.Write.MSGStatus.ErrorCount,1,@91194825@.CONTROL.DPV1.Write.MSGStatus.ErrorCount) ,OTL(@91194825@.CONTROL.DPV1.Write.MSGStatus.Error) ] ] ,[XIC(@91194825@.CONTROL.DPV1.Alarm.Initiate) [MOV(8732,@91194825@.CONTROL.DPV1.Alarm.Request.Command) ,MSG(@5c6c5012@) ,OTU(@91194825@.CONTROL.DPV1.Alarm.Initiate) ,OTU(@91194825@.CONTROL.DPV1.Alarm.MSGStatus.Error) ,OTU(@91194825@.CONTROL.DPV1.Alarm.MSGStatus.Done) ] ,XIC(@5c6c5012@.DN) [XIO(@91194825@.CONTROL.DPV1.Alarm.MSGStatus.Done) ADD(@91194825@.CONTROL.DPV1.Alarm.MSGStatus.DoneCount,1,@91194825@.CONTROL.DPV1.Alarm.MSGStatus.DoneCount) ,OTL(@91194825@.CONTROL.DPV1.Alarm.MSGStatus.Done) ] ,XIC(@5c6c5012@.ER) [XIO(@91194825@.CONTROL.DPV1.Alarm.MSGStatus.Error) ADD(@91194825@.CONTROL.DPV1.Alarm.MSGStatus.ErrorCount,1,@91194825@.CONTROL.DPV1.Alarm.MSGStatus.ErrorCount) ,OTL(@91194825@.CONTROL.DPV1.Alarm.MSGStatus.Error) ] ] ];
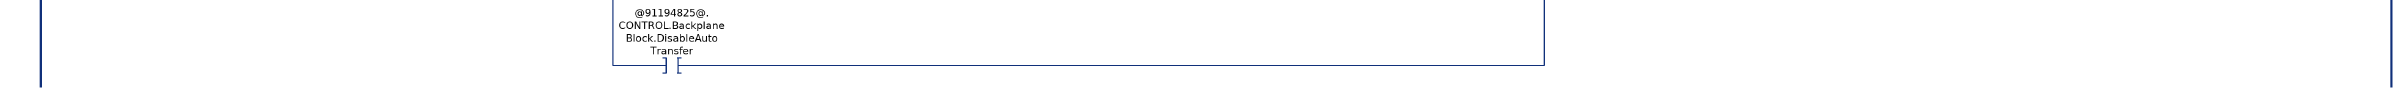
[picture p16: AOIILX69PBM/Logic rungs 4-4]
   // Handle Input Data
   4: [COP(@16b83234@[0],@64f6928d@.InputArray,1) OTU(@624ee698@) ,[[XIC(@64f6928d@.InputArray.DeviceStatusRegister.Communication) XIO(@91194825@.STATUS.Communication) OTL(@91194825@.STATUS.Communication) ,XIO(@64f6928d@.InputArray.DeviceStatusRegister.Communication) XIC(@91194825@.STATUS.Communication) OTU(@91194825@.STATUS.Communication) ] ,[XIC(@64f6928d@.InputArray.DeviceStatusRegister.Running) XIO(@91194825@.STATUS.Running) OTL(@91194825@.STATUS.Running) ,XIO(@64f6928d@.InputArray.DeviceStatusRegister.Running) XIC(@91194825@.STATUS.Running) OTU(@91194825@.STATUS.Running) ] ,[XIC(@64f6928d@.InputArray.DeviceStatusRegister.Ready) XIO(@91194825@.STATUS.Ready) OTL(@91194825@.STATUS.Ready) ,XIO(@64f6928d@.InputArray.DeviceStatusRegister.Ready) XIC(@91194825@.STATUS.Ready) OTU(@91194825@.STATUS.Ready) ] ,COP(@64f6928d@.InputArray.DeviceStatusRegister.BlockTransferOut,@91194825@.STATUS.BackplaneBlock.Output.BlockID,1) COP(@64f6928d@.InputArray.DeviceStatusRegister.BlockTransferIn,@91194825@.STATUS.BackplaneBlock.Input.ReturnedBlockID,1) ] ,COP(@64f6928d@.InputArray.FirmwareRevBPSize,@91194825@.STATUS.FirmwareRevision,1) ,[[XIC(@64f6928d@.InputArray.GlobalStateField.ControlError) XIO(@91194825@.STATUS.GlobalState.ControlError) OTL(@91194825@.STATUS.GlobalState.ControlError) ,XIO(@64f6928d@.InputArray.GlobalStateField.ControlError) XIC(@91194825@.STATUS.GlobalState.ControlError) OTU(@91194825@.STATUS.GlobalState.ControlError) ] ,[XIC(@64f6928d@.InputArray.GlobalStateField.AutoClearError) XIO(@91194825@.STATUS.GlobalState.AutoClearError) OTL(@91194825@.STATUS.GlobalState.AutoClearError) ,XIO(@64f6928d@.InputArray.GlobalStateField.AutoClearError) XIC(@91194825@.STATUS.GlobalState.AutoClearError) OTU(@91194825@.STATUS.GlobalState.AutoClearError) ] ,[XIC(@64f6928d@.InputArray.GlobalStateField.NonExchangeError) XIO(@91194825@.STATUS.GlobalState.NonExchangeError) OTL(@91194825@.STATUS.GlobalState.NonExchangeError) ,XIO(@64f6928d@.InputArray.GlobalStateField.NonExchangeError) XIC(@91194825@.STATUS.GlobalState.NonExchangeError) OTU(@91194825@.STATUS.GlobalState.NonExchangeError) ] ,[XIC(@64f6928d@.InputArray.GlobalStateField.FatalError) XIO(@91194825@.STATUS.GlobalState.FatalError) OTL(@91194825@.STATUS.GlobalState.FatalError) ,XIO(@64f6928d@.InputArray.GlobalStateField.FatalError) XIC(@91194825@.STATUS.GlobalState.FatalError) OTU(@91194825@.STATUS.GlobalState.FatalError) ] ,[XIC(@64f6928d@.InputArray.GlobalStateField.EventError) XIO(@91194825@.STATUS.GlobalState.EventError) OTL(@91194825@.STATUS.GlobalState.EventError) ,XIO(@64f6928d@.InputArray.GlobalStateField.EventError) XIC(@91194825@.STATUS.GlobalState.EventError) OTU(@91194825@.STATUS.GlobalState.EventError) ] ,[XIC(@64f6928d@.InputArray.GlobalStateField.HostNotReady) XIO(@91194825@.STATUS.GlobalState.HostNotReady) OTL(@91194825@.STATUS.GlobalState.HostNotReady) ,XIO(@64f6928d@.InputArray.GlobalStateField.HostNotReady) XIC(@91194825@.STATUS.GlobalState.HostNotReady) OTU(@91194825@.STATUS.GlobalState.HostNotReady) ] ,[XIC(@64f6928d@.InputArray.GlobalStateField.Timeout) XIO(@91194825@.STATUS.GlobalState.Timeout) OTL(@91194825@.STATUS.GlobalState.Timeout) ,XIO(@64f6928d@.InputArray.GlobalStateField.Timeout) XIC(@91194825@.STATUS.GlobalState.Timeout) OTU(@91194825@.STATUS.GlobalState.Timeout) ] ,COP(@64f6928d@.InputArray.GlobalStateField.MasterMainState,@91194825@.STATUS.GlobalState.MasterMainState,7) ,COP(@64f6928d@.InputArray.GlobalStateField.SlaveConfiguration,@91194825@.STATUS.GlobalState.SlaveConfiguration,3) ] ,COP(@64f6928d@.InputArray.SlaveDiagnostic,@91194825@.CONTROL.SlaveDiagnostic.GetSlaveDiag.Response,1) ,[[XIC(@64f6928d@.InputArray.DPV1AlarmIndication.AlarmIndication) XIO(@91194825@.STATUS.DPV1AlarmIndication.AlarmIndication) OTL(@91194825@.STATUS.DPV1AlarmIndication.AlarmIndication) ,XIO(@64f6928d@.InputArray.DPV1AlarmIndication.AlarmIndication) XIC(@91194825@.STATUS.DPV1AlarmIndication.AlarmIndication) OTU(@91194825@.STATUS.DPV1AlarmIndication.AlarmIndication) ] ,[XIC(@64f6928d@.InputArray.DPV1AlarmIndication.AlarmOverrun) XIO(@91194825@.STATUS.DPV1AlarmIndication.AlarmOverrun) OTL(@91194825@.STATUS.DPV1AlarmIndication.AlarmOverrun) ,XIO(@64f6928d@.InputArray.DPV1AlarmIndication.AlarmOverrun) XIC(@91194825@.STATUS.DPV1AlarmIndication.AlarmOverrun) OTU(@91194825@.STATUS.DPV1AlarmIndication.AlarmOverrun) ] ,COP(@64f6928d@.InputArray.DPV1AlarmIndication.AlarmIndicationCounter,@91194825@.STATUS.DPV1AlarmIndication.AlarmIndicationCounter,6) ] ,[SIZE(@16b83234@[0],0,@64f6928d@.InputSize) CPT(@64f6928d@.InputSize,(@64f6928d@.InputSize-44)*2) SIZE(@91194825@.DATA.INPUT[0],0,@64f6928d@.InputDataSize) ,[EQU(@64f6928d@.InputArray.FirmwareRevBPSize.Input,1) MOV(0,@64f6928d@.Config.MaxBlockTransferIn) ,GRT(@64f6928d@.InputArray.FirmwareRevBPSize.Input,1) MOV(@64f6928d@.InputArray.FirmwareRevBPSize.Input,@64f6928d@.Config.MaxBlockTransferIn) ] ,[GRT(@64f6928d@.Config.MaxBlockTransferIn,14) MOV(14,@64f6928d@.Config.MaxBlockTransferIn) ,LES(@64f6928d@.Config.MaxBlockTransferIn,0) MOV(0,@64f6928d@.Config.MaxBlockTransferIn) ] ,[LES(@91194825@.CONTROL.BackplaneBlock.Input.BlockID,0) ,GRT(@91194825@.CONTROL.BackplaneBlock.Input.BlockID,@64f6928d@.Config.MaxBlockTransferIn) ,GRT(@91194825@.CONTROL.BackplaneBlock.Input.BlockID,14) ] MOV(0,@91194825@.CONTROL.BackplaneBlock.Input.BlockID) ,NEQ(@64f6928d@.InputSize,0) [[LES(@64f6928d@.InputSize,408) ,LES(@64f6928d@.InputDataSize,408) ] [LEQ(@64f6928d@.InputSize,@64f6928d@.InputDataSize) MOV(@64f6928d@.InputSize,@64f6928d@.InputCopyLength) ,GRT(@64f6928d@.InputSize,@64f6928d@.InputDataSize) MOV(@64f6928d@.InputDataSize,@64f6928d@.InputCopyLength) ,MOV(0,@64f6928d@.Config.MaxBlockTransferIn) ] ,GEQ(@64f6928d@.InputSize,408) GEQ(@64f6928d@.InputDataSize,408) CPT(@64f6928d@.InputCopyLength,@64f6928d@.InputDataSize MOD @64f6928d@.InputSize) EQU(@64f6928d@.InputCopyLength,0) MOV(@64f6928d@.InputSize,@64f6928d@.InputCopyLength) ] ] ,GRT(@64f6928d@.Config.MaxBlockTransferIn,0) NEQ(@91194825@.CONTROL.BackplaneBlock.Input.BlockID,@64f6928d@.InputArray.DeviceStatusRegister.BlockTransferIn) OTU(@91194825@.STATUS.BackplaneBlock.Input.BlockRead) ,[EQU(@64f6928d@.Config.MaxBlockTransferIn,0) MOV(0,@91194825@.CONTROL.BackplaneBlock.Input.BlockID) MOV(0,@64f6928d@.InputOffset) OTL(@91194825@.STATUS.BackplaneBlock.Input.BlockRead) ,GRT(@64f6928d@.Config.MaxBlockTransferIn,0) EQU(@91194825@.CONTROL.BackplaneBlock.Input.BlockID,@64f6928d@.InputArray.DeviceStatusRegister.BlockTransferIn) [LIM(1,@64f6928d@.InputArray.DeviceStatusRegister.BlockTransferIn,14) SUB(@64f6928d@.InputArray.DeviceStatusRegister.BlockTransferIn,1,@64f6928d@.InputArray.DeviceStatusRegister.BlockTransferIn) CPT(@64f6928d@.InputOffset,@64f6928d@.InputArray.DeviceStatusRegister.BlockTransferIn*@64f6928d@.InputSize) ,XIC(@91194825@.STATUS.Communication) [XIO(@91194825@.CONTROL.BackplaneBlock.DisableAutoTransfer) [LES(@91194825@.CONTROL.BackplaneBlock.Input.BlockID,@64f6928d@.Config.MaxBlockTransferIn) ADD(@91194825@.CONTROL.BackplaneBlock.Input.BlockID,1,@91194825@.CONTROL.BackplaneBlock.Input.BlockID) MOV(408,@64f6928d@.InputCopyLength) OTL(@624ee698@) ,XIO(@624ee698@) EQU(@91194825@.CONTROL.BackplaneBlock.Input.BlockID,@64f6928d@.Config.MaxBlockTransferIn) MOV(0,@91194825@.CONTROL.BackplaneBlock.Input.BlockID) ] ,XIC(@91194825@.CONTROL.BackplaneBlock.DisableAutoTransfer) ] OTL(@91194825@.STATUS.BackplaneBlock.Input.BlockRead) NEQ(@64f6928d@.InputArray.DeviceStatusRegister.BlockTransferIn,0) ] ] LES(@64f6928d@.InputOffset,@64f6928d@.InputDataSize) COP(@64f6928d@.InputArray.InputData[0],@91194825@.DATA.INPUT[@64f6928d@.InputOffset],@64f6928d@.InputCopyLength) ];
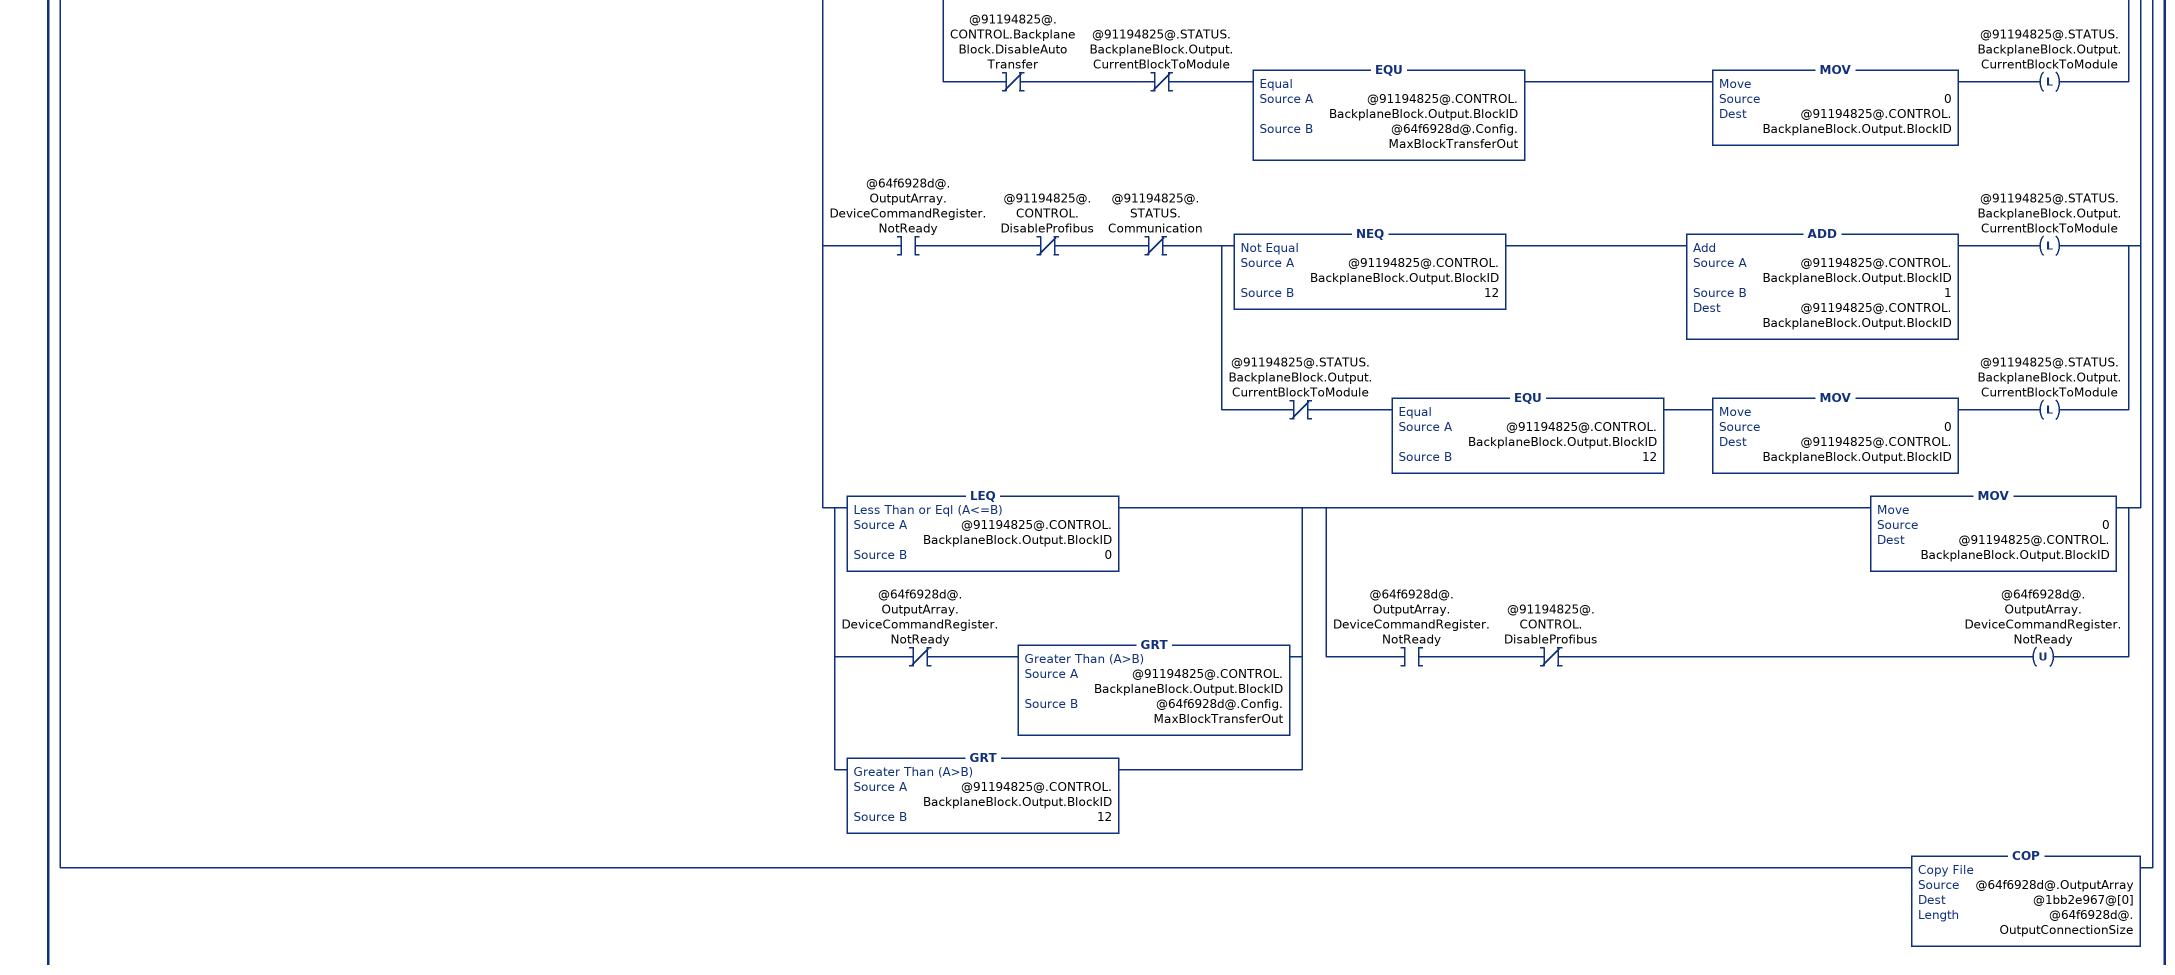
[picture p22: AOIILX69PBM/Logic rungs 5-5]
   // Handle Output Data
   5: [[[[XIC(@91194825@.CONTROL.DisableProfibus) XIO(@64f6928d@.OutputArray.DeviceCommandRegister.NotReady) OTL(@64f6928d@.OutputArray.DeviceCommandRegister.NotReady) ,XIO(@91194825@.CONTROL.DisableProfibus) XIC(@16b83234@[0].6) XIC(@16b83234@[0].7) OTU(@64f6928d@.OutputArray.DeviceCommandRegister.NotReady) ] ,[XIC(@91194825@.CONTROL.ColdBoot) XIO(@64f6928d@.OutputArray.DeviceCommandRegister.Reset) OTL(@64f6928d@.OutputArray.DeviceCommandRegister.Reset) ,XIO(@91194825@.CONTROL.ColdBoot) XIC(@64f6928d@.OutputArray.DeviceCommandRegister.Reset) OTU(@64f6928d@.OutputArray.DeviceCommandRegister.Reset) ] ,[XIO(@91194825@.CONTROL.BackplaneBlock.DisableAutoTransfer) ,XIC(@91194825@.CONTROL.BackplaneBlock.DisableAutoTransfer) [XIC(@91194825@.CONTROL.BackplaneBlock.Output.WriteBlock) ,XIC(@91194825@.CONTROL.BackplaneBlock.Output.CommitToProfibus) MOV(0,@91194825@.CONTROL.BackplaneBlock.Output.BlockID) OTU(@91194825@.CONTROL.BackplaneBlock.Output.CommitToProfibus) ] ] COP(@91194825@.CONTROL.BackplaneBlock.Output.BlockID,@64f6928d@.OutputArray.DeviceCommandRegister.BlockTransferOut,1) OTU(@91194825@.CONTROL.BackplaneBlock.Output.WriteBlock) ,[XIO(@91194825@.CONTROL.BackplaneBlock.DisableAutoTransfer) ,XIC(@91194825@.CONTROL.BackplaneBlock.DisableAutoTransfer) XIC(@91194825@.CONTROL.BackplaneBlock.Input.ReadBlock) ] COP(@91194825@.CONTROL.BackplaneBlock.Input.BlockID,@64f6928d@.OutputArray.DeviceCommandRegister.BlockTransferIn,1) OTU(@91194825@.CONTROL.BackplaneBlock.Input.ReadBlock) ] ,MOV(@91194825@.CONTROL.SlaveDiagnostic.GetSlaveDiag.Address,@64f6928d@.OutputArray.DiagnosticSlaveAddress.SlaveAddress) MOV(@91194825@.CONTROL.SlaveDiagnostic.GetSlaveDiag.Function,@64f6928d@.OutputArray.DiagnosticSlaveAddress.DiagnosticMode) ,[MOV(@91194825@.CONTROL.SlaveControl.SetSlaveControl.Address,@64f6928d@.OutputArray.GlobalControlCommand.SlaveAddress) ,[XIC(@91194825@.CONTROL.SlaveControl.SetSlaveControl.SlaveCommand.ClearData) XIO(@64f6928d@.OutputArray.GlobalControlCommand.ControlCommand.1) OTL(@64f6928d@.OutputArray.GlobalControlCommand.ControlCommand.1) ,XIO(@91194825@.CONTROL.SlaveControl.SetSlaveControl.SlaveCommand.ClearData) XIC(@64f6928d@.OutputArray.GlobalControlCommand.ControlCommand.1) OTU(@64f6928d@.OutputArray.GlobalControlCommand.ControlCommand.1) ] ,[XIC(@91194825@.CONTROL.SlaveControl.SetSlaveControl.SlaveCommand.UnFreeze) XIO(@64f6928d@.OutputArray.GlobalControlCommand.ControlCommand.2) OTL(@64f6928d@.OutputArray.GlobalControlCommand.ControlCommand.2) ,XIO(@91194825@.CONTROL.SlaveControl.SetSlaveControl.SlaveCommand.UnFreeze) XIC(@64f6928d@.OutputArray.GlobalControlCommand.ControlCommand.2) OTU(@64f6928d@.OutputArray.GlobalControlCommand.ControlCommand.2) ] ,[XIC(@91194825@.CONTROL.SlaveControl.SetSlaveControl.SlaveCommand.Freeze) XIO(@64f6928d@.OutputArray.GlobalControlCommand.ControlCommand.3) OTL(@64f6928d@.OutputArray.GlobalControlCommand.ControlCommand.3) ,XIO(@91194825@.CONTROL.SlaveControl.SetSlaveControl.SlaveCommand.Freeze) XIC(@64f6928d@.OutputArray.GlobalControlCommand.ControlCommand.3) OTU(@64f6928d@.OutputArray.GlobalControlCommand.ControlCommand.3) ] ,[XIC(@91194825@.CONTROL.SlaveControl.SetSlaveControl.SlaveCommand.UnSync) XIO(@64f6928d@.OutputArray.GlobalControlCommand.ControlCommand.4) OTL(@64f6928d@.OutputArray.GlobalControlCommand.ControlCommand.4) ,XIO(@91194825@.CONTROL.SlaveControl.SetSlaveControl.SlaveCommand.UnSync) XIC(@64f6928d@.OutputArray.GlobalControlCommand.ControlCommand.4) OTU(@64f6928d@.OutputArray.GlobalControlCommand.ControlCommand.4) ] ,[XIC(@91194825@.CONTROL.SlaveControl.SetSlaveControl.SlaveCommand.Sync) XIO(@64f6928d@.OutputArray.GlobalControlCommand.ControlCommand.5) OTL(@64f6928d@.OutputArray.GlobalControlCommand.ControlCommand.5) ,XIO(@91194825@.CONTROL.SlaveControl.SetSlaveControl.SlaveCommand.Sync) XIC(@64f6928d@.OutputArray.GlobalControlCommand.ControlCommand.5) OTU(@64f6928d@.OutputArray.GlobalControlCommand.ControlCommand.5) ] ,MOV(@91194825@.CONTROL.SlaveControl.SetSlaveControl.SlaveCommand.GroupSelect,@64f6928d@.OutputArray.GlobalControlCommand.GroupSelect) ] ] ,[SIZE(@1bb2e967@[0],0,@64f6928d@.OutputConnectionSize) CPT(@64f6928d@.OutputSize,@64f6928d@.OutputConnectionSize-8) SIZE(@64f6928d@.OutputArray.OutputData[0],0,@64f6928d@.UTILOutputCopyLength) SIZE(@91194825@.DATA.OUTPUT[0],0,@64f6928d@.OutputDataSize) DIV(@64f6928d@.OutputDataSize,2,@64f6928d@.OutputDataSize) ,[[EQU(@64f6928d@.InputArray.FirmwareRevBPSize.Output,1) MOV(0,@64f6928d@.Config.MaxBlockTransferOut) ,GRT(@64f6928d@.InputArray.FirmwareRevBPSize.Output,1) MOV(@64f6928d@.InputArray.FirmwareRevBPSize.Output,@64f6928d@.Config.MaxBlockTransferOut) ] ,GRT(@64f6928d@.Config.MaxBlockTransferOut,12) MOV(12,@64f6928d@.Config.MaxBlockTransferOut) ,LES(@64f6928d@.Config.MaxBlockTransferOut,0) MOV(0,@64f6928d@.Config.MaxBlockTransferOut) ] ,[[LES(@64f6928d@.OutputSize,240) ,LES(@64f6928d@.OutputDataSize,240) ] [LEQ(@64f6928d@.OutputSize,@64f6928d@.OutputDataSize) MOV(@64f6928d@.OutputSize,@64f6928d@.OutputCopyLastLength) ,GRT(@64f6928d@.OutputSize,@64f6928d@.OutputDataSize) MOV(@64f6928d@.OutputDataSize,@64f6928d@.OutputCopyLastLength) ,XIO(@64f6928d@.OutputArray.DeviceCommandRegister.NotReady) MOV(0,@64f6928d@.Config.MaxBlockTransferOut) ] ,GEQ(@64f6928d@.OutputDataSize,240) GEQ(@64f6928d@.OutputSize,240) CPT(@64f6928d@.OutputCopyLastLength,@64f6928d@.OutputDataSize MOD @64f6928d@.OutputSize) XIO(@64f6928d@.OutputArray.DeviceCommandRegister.NotReady) CPT(@64f6928d@.Config.MaxBlockDataOut,@64f6928d@.OutputDataSize / @64f6928d@.OutputSize + 1) [EQU(@64f6928d@.OutputCopyLastLength,0) [SUB(@64f6928d@.Config.MaxBlockDataOut,1,@64f6928d@.Config.MaxBlockDataOut) ,MOV(@64f6928d@.OutputSize,@64f6928d@.OutputCopyLastLength) ] ,LES(@64f6928d@.Config.MaxBlockDataOut,@64f6928d@.Config.MaxBlockTransferOut) MOV(@64f6928d@.Config.MaxBlockDataOut,@64f6928d@.Config.MaxBlockTransferOut) ] ] ,[LES(@91194825@.CONTROL.BackplaneBlock.Output.BlockID,0) ,XIO(@64f6928d@.OutputArray.DeviceCommandRegister.NotReady) [GRT(@91194825@.CONTROL.BackplaneBlock.Output.BlockID,@64f6928d@.Config.MaxBlockTransferOut) ,EQU(0,@64f6928d@.Config.MaxBlockTransferOut) ] ,GRT(@91194825@.CONTROL.BackplaneBlock.Output.BlockID,12) ] [MOV(0,@91194825@.CONTROL.BackplaneBlock.Output.BlockID) ,XIC(@64f6928d@.OutputArray.DeviceCommandRegister.NotReady) XIO(@91194825@.CONTROL.DisableProfibus) OTU(@64f6928d@.OutputArray.DeviceCommandRegister.NotReady) ] ] ,[EQU(@64f6928d@.Config.MaxBlockTransferOut,0) [MOV(0,@64f6928d@.OutputOffset) ,MOV(@64f6928d@.OutputCopyLastLength,@64f6928d@.OutputCopyLength) ] OTL(@91194825@.STATUS.BackplaneBlock.Output.CommittedToProfibus) OTL(@91194825@.STATUS.BackplaneBlock.Output.CurrentBlockToModule) FLL(0,@64f6928d@.OutputArray.OutputData[0],@64f6928d@.UTILOutputCopyLength) ,GRT(@64f6928d@.Config.MaxBlockTransferOut,0) NEQ(@91194825@.CONTROL.BackplaneBlock.Output.BlockID,@64f6928d@.InputArray.DeviceStatusRegister.BlockTransferOut) [NEQ(@91194825@.CONTROL.BackplaneBlock.Output.BlockID,0) OTU(@91194825@.STATUS.BackplaneBlock.Output.CommittedToProfibus) ,NEQ(@91194825@.CONTROL.BackplaneBlock.Output.BlockID,@64f6928d@.Config.MaxBlockTransferOut) MOV(@64f6928d@.OutputSize,@64f6928d@.OutputCopyLength) ,EQU(@91194825@.CONTROL.BackplaneBlock.Output.BlockID,@64f6928d@.Config.MaxBlockTransferOut) MOV(@64f6928d@.OutputCopyLastLength,@64f6928d@.OutputCopyLength) ,OTU(@91194825@.STATUS.BackplaneBlock.Output.CurrentBlockToModule) ,CPT(@64f6928d@.OutputOffset,(@64f6928d@.OutputArray.DeviceCommandRegister.BlockTransferOut-1)*@64f6928d@.OutputSize*2) ] ] GEQ(@64f6928d@.OutputOffset,0) CMP(@64f6928d@.OutputOffset<@64f6928d@.OutputDataSize*2) COP(@91194825@.DATA.OUTPUT[@64f6928d@.OutputOffset],@64f6928d@.OutputArray.OutputData[0],@64f6928d@.OutputCopyLength) ,GRT(@64f6928d@.Config.MaxBlockTransferOut,0) EQU(@91194825@.CONTROL.BackplaneBlock.Output.BlockID,@64f6928d@.InputArray.DeviceStatusRegister.BlockTransferOut) XIC(@91194825@.STATUS.Running) XIC(@91194825@.STATUS.Ready) [XIC(@91194825@.STATUS.Communication) [EQU(@64f6928d@.InputArray.DeviceStatusRegister.BlockTransferOut,0) OTL(@91194825@.STATUS.BackplaneBlock.Output.CommittedToProfibus) ,[XIO(@91194825@.CONTROL.BackplaneBlock.DisableAutoTransfer) NEQ(@91194825@.CONTROL.BackplaneBlock.Output.BlockID,@64f6928d@.Config.MaxBlockTransferOut) ADD(@91194825@.CONTROL.BackplaneBlock.Output.BlockID,1,@91194825@.CONTROL.BackplaneBlock.Output.BlockID) ,XIC(@91194825@.CONTROL.BackplaneBlock.DisableAutoTransfer) ] OTL(@91194825@.STATUS.BackplaneBlock.Output.CurrentBlockToModule) ,XIO(@91194825@.CONTROL.BackplaneBlock.DisableAutoTransfer) XIO(@91194825@.STATUS.BackplaneBlock.Output.CurrentBlockToModule) EQU(@91194825@.CONTROL.BackplaneBlock.Output.BlockID,@64f6928d@.Config.MaxBlockTransferOut) MOV(0,@91194825@.CONTROL.BackplaneBlock.Output.BlockID) OTL(@91194825@.STATUS.BackplaneBlock.Output.CurrentBlockToModule) ] ,XIC(@64f6928d@.OutputArray.DeviceCommandRegister.NotReady) XIO(@91194825@.CONTROL.DisableProfibus) XIO(@91194825@.STATUS.Communication) [NEQ(@91194825@.CONTROL.BackplaneBlock.Output.BlockID,12) ADD(@91194825@.CONTROL.BackplaneBlock.Output.BlockID,1,@91194825@.CONTROL.BackplaneBlock.Output.BlockID) OTL(@91194825@.STATUS.BackplaneBlock.Output.CurrentBlockToModule) ,XIO(@91194825@.STATUS.BackplaneBlock.Output.CurrentBlockToModule) EQU(@91194825@.CONTROL.BackplaneBlock.Output.BlockID,12) MOV(0,@91194825@.CONTROL.BackplaneBlock.Output.BlockID) OTL(@91194825@.STATUS.BackplaneBlock.Output.CurrentBlockToModule) ] ,[LEQ(@91194825@.CONTROL.BackplaneBlock.Output.BlockID,0) ,XIO(@64f6928d@.OutputArray.DeviceCommandRegister.NotReady) GRT(@91194825@.CONTROL.BackplaneBlock.Output.BlockID,@64f6928d@.Config.MaxBlockTransferOut) ,GRT(@91194825@.CONTROL.BackplaneBlock.Output.BlockID,12) ] [MOV(0,@91194825@.CONTROL.BackplaneBlock.Output.BlockID) ,XIC(@64f6928d@.OutputArray.DeviceCommandRegister.NotReady) XIO(@91194825@.CONTROL.DisableProfibus) OTU(@64f6928d@.OutputArray.DeviceCommandRegister.NotReady) ] ] ,COP(@64f6928d@.OutputArray,@1bb2e967@[0],@64f6928d@.OutputConnectionSize) ];
END_ROUTINE

ROUTINE Prescan   (* ladder *)
// Prescan
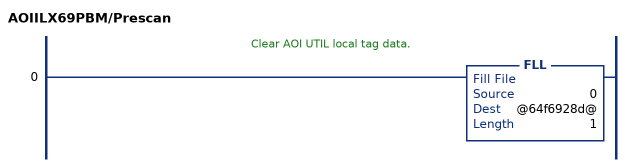
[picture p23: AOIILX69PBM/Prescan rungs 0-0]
   // Clear AOI UTIL local tag data.
   0: FLL(0,@64f6928d@,1);
END_ROUTINE
END_ADD_ON_INSTRUCTION

VAR_GLOBAL   (* controller tags *)
   ILX69PBM_MSGDPV1Read : MESSAGE;   // DPV1 Read Message
        MessageParameters(MessageType := CIP Generic, RequestedLength := 12, ConnectedFlag := 2, ConnectionPath := PBM, ServiceCode := 16#0064, ObjectType := 16#0065, TargetObject := 1, LocalElement := ILX69PBM.CONTROL.DPV1.Read.Request, DestinationTag := ILX69PBM.CONTROL.DPV1.Read.Response)
   ILX69PBM_MSGDPV1Write : MESSAGE;   // DPV1 Write Message
        MessageParameters(MessageType := CIP Generic, RequestedLength := 22, ConnectedFlag := 2, ConnectionPath := PBM, ServiceCode := 16#0064, ObjectType := 16#0065, TargetObject := 1, LocalElement := ILX69PBM.CONTROL.DPV1.Write.Request, DestinationTag := ILX69PBM.CONTROL.DPV1.Write.Response)
   Local:1:I : AB:1769_MODULE_INT_500Bytes:I:0;
   ILX69PBM_MSGSlaveControl : MESSAGE;   // Slave Control Message
        MessageParameters(MessageType := CIP Generic, RequestedLength := 24, ConnectedFlag := 2, ConnectionPath := PBM, ServiceCode := 16#0064, ObjectType := 16#0065, TargetObject := 1, LocalElement := ILX69PBM.CONTROL.SlaveControl.SetSlaveControl_MSG.Request, DestinationTag := ILX69PBM.CONTROL.SlaveControl.SetSlaveControl_MSG.Response)
   ILX69PBM_MSGSlaveDiagRequest : MESSAGE;   // Slave Diagnostic Request Message
        MessageParameters(MessageType := CIP Generic, RequestedLength := 16, ConnectedFlag := 2, ConnectionPath := PBM, ServiceCode := 16#0064, ObjectType := 16#0065, TargetObject := 1, LocalElement := ILX69PBM.CONTROL.SlaveDiagnostic.GetSlaveDiagExtended_MSG.Request, DestinationTag := ILX69PBM.CONTROL.SlaveDiagnostic.GetSlaveDiagExtended_MSG.Response)
   Local:1:O : AB:1769_MODULE_INT_496Bytes:O:0;
   ILX69PBM_MSGDPV1Alarm : MESSAGE;   // DPV1 Alarm Response Message
        MessageParameters(MessageType := CIP Generic, RequestedLength := 16, ConnectedFlag := 2, ConnectionPath := PBM, ServiceCode := 16#0064, ObjectType := 16#0065, TargetObject := 1, LocalElement := ILX69PBM.CONTROL.DPV1.Alarm.Request, DestinationTag := ILX69PBM.CONTROL.DPV1.Alarm.Response)
   AOIILX69PBM : AOIILX69PBM;
   ILX69PBM : ILX69PBM_MODULEDEF;
END_VAR

PROGRAM MainProgram

ROUTINE MainRoutine   (* ladder *)
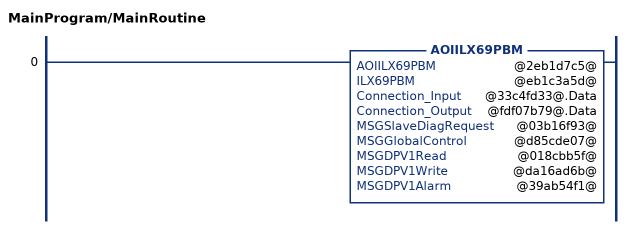
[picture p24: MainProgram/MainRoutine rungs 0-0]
   0: AOIILX69PBM(@2eb1d7c5@,@eb1c3a5d@,@33c4fd33@.Data,@fdf07b79@.Data,@03b16f93@,@d85cde07@,@018cbb5f@,@da16ad6b@,@39ab54f1@);
END_ROUTINE
END_PROGRAM
